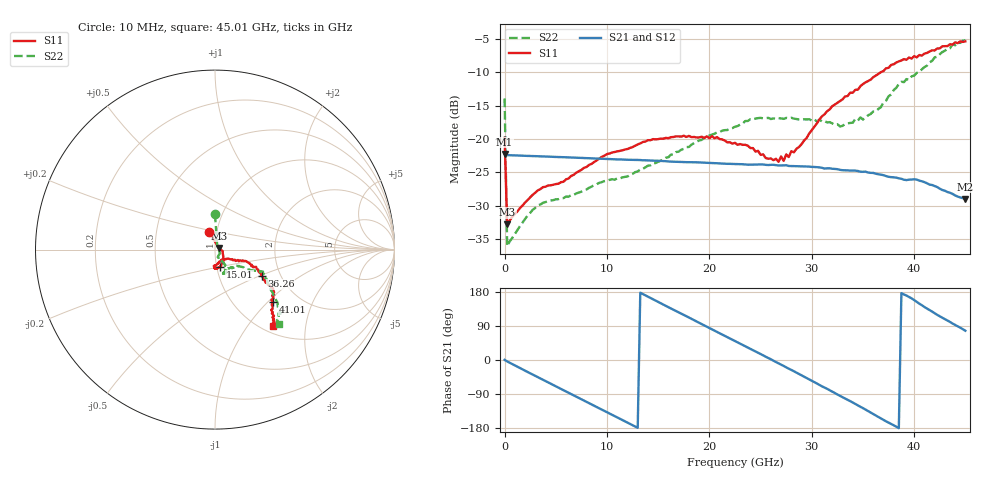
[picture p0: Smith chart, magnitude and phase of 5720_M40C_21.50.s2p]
! Device:  ADRF5720
! Description: 0.5dB LSB GaAs MMIC 6-bit Digital Attenuator
! Frequency:  0.000009 -  40 GHz
! Ports:
!	RF1	= Port 1
!	RF2	= Port 2
! Vdd:  3.3 Volt
! Vss:  -3.3 Volt
! Control:  0/3.3 Volt
! State:  21.50 dB attenuation
! Data:  The device was measured using G-S-G Probes on a matrix board.
!  Data was collected using an calibrated 4 port network analyzer.
!  The reference plane for this measurement is at the launchers.
! Note:  Analog Devices supplies this data as a sample of measured data
!  for this product.  Your particular data for this product may vary.
!  Data was taken at -40 degrees C.
!  Analog Devices reserves the right to change this data at anytime.
# GHZ S DB R 45.0
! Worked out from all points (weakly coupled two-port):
!   181 points, 10 MHz to 45.01 GHz, reference 45 ohm
!   highest |S21| = -22.24 dB at 10 MHz (marker M1); lowest = -29.0 dB at 45.01 GHz (marker M2)
!   lowest |S11| = -32.7 dB at 260 MHz (marker M3), VSWR 1.05, Z = 46.9 + j0.88 ohm
!   |S11| at or under -10 dB: start of sweep to 36.76 GHz
!   |S22| runs from -36.0 to -5.3 dB; largest |S21 - S12| = 0.00028
!   S11 on the Smith chart (normalised r, x): 10 MHz: 0.92, +0.18; 15.01 GHz: 1.04, -0.20; 36.26 GHz: 1.60, -0.51; 41.01 GHz: 1.49, -1.07; 45.01 GHz: 1.11, -1.34
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0.01  -19.83 108.7  -22.24 0.4  -22.26 0.4  -13.94 90.1
0.26  -32.74 24.0  -22.42 -3.8  -22.44 -3.8  -36.04 31.3
3.26  -27.68 -9.8  -22.59 -45.4  -22.61 -45.5  -29.94 -32.5
7.76  -24.33 -40.5  -22.85 -107.0  -22.87 -107.0  -27.68 -65.6
10.01  -22.26 -51.5  -22.99 -137.8  -23.01 -137.9  -26.21 -68.0
15.01  -20.02 -74.3  -23.26 153.3  -23.28 153.2  -23.41 -60.4
15.26  -19.94 -75.6  -23.28 149.7  -23.30 149.7  -23.26 -60.5
20.26  -19.58 -91.2  -23.60 80.9  -23.62 80.8  -19.35 -57.4
22.76  -20.87 -93.9  -23.76 46.7  -23.79 46.6  -18.07 -62.8
24.01  -21.36 -84.9  -23.85 29.8  -23.87 29.7  -17.05 -64.2
25.51  -22.85 -71.3  -23.87 8.6  -23.89 8.5  -16.89 -65.8
26.76  -23.41 -57.8  -23.96 -8.8  -23.98 -8.9  -16.88 -67.5
27.01  -22.62 -54.5  -23.96 -12.0  -23.98 -12.2  -16.93 -69.4
27.26  -23.28 -53.5  -23.95 -15.7  -23.97 -15.8  -16.99 -68.3
30.26  -18.17 -27.0  -24.19 -58.3  -24.22 -58.5  -17.07 -69.8
32.76  -14.33 -20.8  -24.62 -94.5  -24.64 -94.6  -18.12 -59.0
36.26  -10.52 -29.5  -25.20 -146.5  -25.22 -146.6  -15.88 -34.3
37.76  -8.92 -33.5  -25.71 -168.7  -25.73 -168.9  -13.35 -30.8
39.76  -7.97 -36.6  -26.07 162.5  -26.09 162.3  -10.63 -24.6
41.01  -7.23 -42.0  -26.46 139.9  -26.50 139.7  -9.24 -32.3
43.76  -5.88 -49.8  -28.22 96.1  -28.23 95.9  -5.83 -44.3
45.01  -5.40 -52.8  -28.97 77.2  -28.99 77.1  -5.26 -49.6
